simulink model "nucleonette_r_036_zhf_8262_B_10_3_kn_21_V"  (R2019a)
settings: Solver=VariableStepAuto  StartTime=0.0  StopTime=727544.216  FixedStep=0.2  RelTol=1e-6
libraries: simulink x6
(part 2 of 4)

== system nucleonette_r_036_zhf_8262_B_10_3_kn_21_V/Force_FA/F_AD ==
  In1 : Inport
  In2 : Inport  Port=2
  Add21 : Sum  Inputs=+-
  Add27 : Sum  Inputs=-+++
  Add32 : Sum  Inputs=+++
  Add35 : Sum
  Add38 : Sum  Inputs=++++
  Add53 : Sum
  C_100_1 : Constant  Value=-100
  C_10_1 : Constant  Value=10
  C_10_11_2 : Constant  Value=1E-21
  Clock1 : Clock
  Constant : Constant
  Constant1 : Constant  Value=2
  Constant13 : Constant  Value=3
  Constant15 : Constant  Value=1.0E-3
  Constant19 : Constant  Value=2
  Constant24 : Constant  Value=3
  Constant26 : Constant  Value=3
  Math Function{17,24,34,36} (4 alike) : Math  Operator=square
  Math Function35 : Math  Operator=pow
  Math Function39 : Math  Operator=pow
  Math Function45 : Math  Operator=pow
  Nadx/Dadx : Scope
  Omega_w1 : Constant  Value=0.00003453723537
  Product{1..4,27,54..56,66} (9 alike) : Product  Inputs=**
  Product{29,46,50,57} (4 alike) : Product
  Product40 : Product  Inputs=*/
  Product48 : Product  Inputs=/**
  Product5 : Product  Inputs=/*
  Product62 : Product  Inputs=*/
  Product63 : Product  Inputs=/*
  Product65 : Product  Inputs=*/*
  Sqrt10 : Sqrt
  Sqrt14 : Sqrt
  Trigonometric Function11 : Trigonometry
  Trigonometric Function12 : Trigonometry  Operator=cos
  Trigonometric Function7 : Trigonometry
  Trigonometric Function8 : Trigonometry  Operator=cos
  ex : Constant  Value=1.602176565
  kADx : Constant  Value=66.535517341
  mFAx : Constant  Value=999.755388642
  rx1 : Constant  Value=0.36373
  Out1 : Outport
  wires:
  Product57/1 -> Trigonometric Function12/1, Product29/2, Trigonometric Function11/1
  Math Function34/1 -> Add32/3  "Zad_2"
  kADx/1 -> Product48/3
  rx1/1 -> Product27/1, Product5/2, Product54/1, Product4/1, Product65/2, Product56/1, Product55/1  "rx"
  In2/1 -> Product1/1  "z4"
  Math Function17/1 -> Add32/1  "Yad_2"
  C_10_11_2/1 -> Add35/2
  Product40/1 -> Nadx/Dadx/1, Out1/1  "nad/dad"
  Omega_w1/1 -> Product57/2
  Add32/1 -> Sqrt10/1  "Dad_2"
  Constant13/1 -> Product29/1, Sqrt14/1
  Product66/1 -> Product50/2  "kn_Dad"
  Add53/1 -> Product40/2  "Dad_B"
  Math Function36/1 -> Add32/2  "Xad_2"
  Product54/1 -> Add21/1  "r*cos(3wt)"
  Product63/1 -> Product3/2, Product1/2  "1/2"
  Add38/1 -> Math Function17/1  "YAD"
  Add27/1 -> Math Function34/1, Product50/1  "ZAD"
  C_10_1/1 -> Math Function39/1
  Product65/1 -> Math Function39/2
  Product29/1 -> Trigonometric Function8/1, Trigonometric Function7/1
  Product62/1 -> Add38/1  "r*sin(3wt)/2"
  Constant1/1 -> Product63/1
  Product50/1 -> Product40/1  "Nad"
  Math Function39/1 -> Add35/1  "10_exp(-100Dad/r)"
  Constant24/1 -> Math Function45/2
  Math Function45/1 -> Add53/1
  Add21/1 -> Math Function36/1  "XAD"
  In1/1 -> Add27/2  "z0 - z + delta"
  ex/1 -> Math Function24/1
  Constant19/1 -> Product62/2, Product5/1  "2"
  Math Function24/1 -> Product48/2
  Sqrt10/1 -> Product65/1, Math Function35/1  "Dad"
  Constant/1 -> Product63/2
  Trigonometric Function11/1 -> Product55/2  "sin(wt)"
  Trigonometric Function12/1 -> Product56/2  "cos(wt)"
  Product2/1 -> Add38/3  "z4*sqrt(3)/2"
  Add35/1 -> Product66/1
  Constant26/1 -> Math Function35/2
  Clock1/1 -> Product57/1
  Product27/1 -> Product46/1, Product62/1  "r*sin(3wt)"
  Product48/1 -> Product66/2
  Math Function35/1 -> Add53/2  "Dad_3"
  Sqrt14/1 -> Product3/1, Product2/1  "sqrt(3)"
  mFAx/1 -> Product48/1  "mx"
  Constant15/1 -> Math Function45/1
  C_100_1/1 -> Product65/3
  Product56/1 -> Add21/2  "r*cos(wt)"
  Trigonometric Function8/1 -> Product54/2  "cos(3wt)"
  Product3/1 -> Product46/2, Product4/2  "sqrt(3)/2"
  Trigonometric Function7/1 -> Product27/2  "sin(3wt)"
  Product5/1 -> Add38/2  "r/2"
  Product1/1 -> Product2/2, Add27/3  "z4/2"
  Product4/1 -> Add27/4  "r*sqrt(3)/2"
  Product55/1 -> Add38/4  "r*sin(wt)"
  Product46/1 -> Add27/1  "r*sin(3wt)*sqrt(3)/2"

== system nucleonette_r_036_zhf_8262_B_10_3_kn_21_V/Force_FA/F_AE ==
  In1 : Inport
  In2 : Inport  Port=2
  Add21 : Sum  Inputs=--
  Add27 : Sum  Inputs=++++
  Add32 : Sum  Inputs=+++
  Add35 : Sum
  Add38 : Sum  Inputs=-+++
  Add53 : Sum
  C_100_1 : Constant  Value=-100
  C_10_1 : Constant  Value=10
  C_10_11_2 : Constant  Value=1E-21
  Clock1 : Clock
  Constant : Constant
  Constant1 : Constant  Value=2
  Constant13 : Constant  Value=3
  Constant15 : Constant  Value=1.0E-3
  Constant19 : Constant  Value=2
  Constant24 : Constant  Value=3
  Constant26 : Constant  Value=3
  Math Function{17,24,34,36} (4 alike) : Math  Operator=square
  Math Function35 : Math  Operator=pow
  Math Function39 : Math  Operator=pow
  Math Function45 : Math  Operator=pow
  Naex/Daex : Scope
  Omega_w1 : Constant  Value=0.00003453723537
  Product{1..4,27,54..56,66} (9 alike) : Product  Inputs=**
  Product{29,46,50,57} (4 alike) : Product
  Product40 : Product  Inputs=*/
  Product48 : Product  Inputs=/**
  Product5 : Product  Inputs=/*
  Product62 : Product  Inputs=*/
  Product63 : Product  Inputs=/*
  Product65 : Product  Inputs=*/*
  Sqrt10 : Sqrt
  Sqrt14 : Sqrt
  Trigonometric Function11 : Trigonometry
  Trigonometric Function12 : Trigonometry  Operator=cos
  Trigonometric Function7 : Trigonometry
  Trigonometric Function8 : Trigonometry  Operator=cos
  ex : Constant  Value=1.602176565
  kAEx : Constant  Value=66.535517341
  mFAx : Constant  Value=999.755388642
  rx1 : Constant  Value=0.36373
  Out1 : Outport
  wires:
  Add38/1 -> Math Function17/1  "YAE"
  Math Function36/1 -> Add32/2  "Xae_2"
  mFAx/1 -> Product48/1  "mx"
  Constant15/1 -> Math Function45/1
  C_100_1/1 -> Product65/3
  Sqrt14/1 -> Product3/1, Product2/1  "sqrt(3)"
  Product55/1 -> Add38/4  "r*sin(wt)"
  Product4/1 -> Add27/4  "r*sqrt(3)/2"
  Math Function39/1 -> Add35/1  "10_exp(-100Dae/r)"
  Constant1/1 -> Product63/1
  Product50/1 -> Product40/1  "Nae"
  Product54/1 -> Add21/1  "r*cos(3wt)"
  Product3/1 -> Product46/2, Product4/2  "sqrt(3)/2"
  Product48/1 -> Product66/2
  Product1/1 -> Product2/2, Add27/3  "z4/2"
  In1/1 -> Add27/2  "z0 - z + delta"
  Add21/1 -> Math Function36/1  "XAE"
  Trigonometric Function11/1 -> Product55/2  "sin(wt)"
  Add35/1 -> Product66/1
  Math Function35/1 -> Add53/2  "Dae_3"
  Trigonometric Function8/1 -> Product54/2  "cos(3wt)"
  Math Function24/1 -> Product48/2
  Product56/1 -> Add21/2  "r*cos(wt)"
  Trigonometric Function7/1 -> Product27/2  "sin(3wt)"
  Constant19/1 -> Product62/2, Product5/1  "2"
  Constant/1 -> Product63/2
  Product2/1 -> Add38/3  "z4*sqrt(3)/2"
  Trigonometric Function12/1 -> Product56/2  "cos(wt)"
  Clock1/1 -> Product57/1
  Constant26/1 -> Math Function35/2
  Product29/1 -> Trigonometric Function8/1, Trigonometric Function7/1
  Product46/1 -> Add27/1  "r*sin(3wt)*sqrt(3)/2"
  Product65/1 -> Math Function39/2
  C_10_1/1 -> Math Function39/1
  Constant24/1 -> Math Function45/2
  ex/1 -> Math Function24/1
  Product57/1 -> Trigonometric Function12/1, Product29/2, Trigonometric Function11/1
  Math Function34/1 -> Add32/3  "Zae_2"
  Product63/1 -> Product3/2, Product1/2  "1/2"
  Product5/1 -> Add38/2  "r/2"
  Add27/1 -> Math Function34/1, Product50/1  "ZAE"
  Omega_w1/1 -> Product57/2
  Constant13/1 -> Product29/1, Sqrt14/1
  Add32/1 -> Sqrt10/1  "Dae_2"
  Product40/1 -> Naex/Daex/1, Out1/1  "nae/dae"
  Product27/1 -> Product46/1, Product62/1  "r*sin(3wt)"
  Math Function45/1 -> Add53/1
  Product66/1 -> Product50/2  "kn_Dae"
  Product62/1 -> Add38/1  "r*sin(3wt)/2"
  kAEx/1 -> Product48/3
  Add53/1 -> Product40/2  "Dae_B"
  rx1/1 -> Product27/1, Product5/2, Product54/1, Product4/1, Product65/2, Product56/1, Product55/1  "rx"
  Sqrt10/1 -> Product65/1, Math Function35/1  "Dae"
  C_10_11_2/1 -> Add35/2
  Math Function17/1 -> Add32/1  "Yae_2"
  In2/1 -> Product1/1  "z4"

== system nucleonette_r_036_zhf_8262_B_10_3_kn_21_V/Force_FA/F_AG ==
  In1 : Inport
  In2 : Inport  Port=2
  Add28 : Sum  Inputs=+-
  Add29 : Sum  Inputs=-++
  Add30 : Sum  Inputs=+++
  Add34 : Sum  Inputs=+++
  Add36 : Sum
  Add54 : Sum
  C_100_1 : Constant  Value=-100
  C_10_1 : Constant  Value=10
  C_10_11_2 : Constant  Value=1E-21
  Clock1 : Clock
  Constant{13,24..26} (4 alike) : Constant  Value=3
  Constant15 : Constant  Value=1.0E-3
  Constant19 : Constant  Value=2
  Constant23 : Constant  Value=2
  Math Function{21,24,26,31} (4 alike) : Math  Operator=square
  Math Function23 : Math  Operator=pow
  Math Function40 : Math  Operator=pow
  Math Function45 : Math  Operator=pow
  Nagx/Dagx_3 : Scope
  Omega_w1 : Constant  Value=0.00003453723537
  Product{27,55..56,62,67} (5 alike) : Product  Inputs=**
  Product{29,46,52,57} (4 alike) : Product
  Product47 : Product  Inputs=*/
  Product48 : Product  Inputs=/**
  Product54 : Product  Inputs=**/
  Product63 : Product  Inputs=/*
  Product64 : Product  Inputs=*/*
  Sqrt13 : Sqrt
  Sqrt14 : Sqrt
  Sqrt15 : Sqrt
  Trigonometric Function11 : Trigonometry
  Trigonometric Function12 : Trigonometry  Operator=cos
  Trigonometric Function7 : Trigonometry
  Trigonometric Function8 : Trigonometry  Operator=cos
  ex : Constant  Value=1.602176565
  k16x1 : Constant  Value=66.535517341
  mFAx : Constant  Value=999.755388642
  rx1 : Constant  Value=0.36373
  Out1 : Outport
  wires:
  Product52/1 -> Product47/1  "Nag"
  Product29/1 -> Trigonometric Function8/1, Trigonometric Function7/1
  C_10_11_2/1 -> Add36/1
  Constant13/1 -> Sqrt13/1
  Add54/1 -> Product47/2  "Dag_B"
  Constant15/1 -> Math Function45/1
  Add29/1 -> Math Function21/1  "X3a"
  Constant25/1 -> Sqrt14/1, Product29/2
  Add34/1 -> Sqrt15/1  "Dag_2"
  Constant24/1 -> Math Function45/2
  Trigonometric Function11/1 -> Product55/2  "sin(wt)"
  Product54/1 -> Add29/3, Product46/1  "r*cos(3wt)/2"
  Constant23/1 -> Product54/3
  Product48/1 -> Product67/2
  Trigonometric Function12/1 -> Product56/2  "cos(wt)"
  Math Function40/1 -> Add36/2  "10_exp(-100Dag/r)"
  Product64/1 -> Math Function40/2
  Trigonometric Function7/1 -> Product27/2  "sin(3wt)"
  Product47/1 -> Out1/1, Nagx/Dagx_3/1  "Nag/Dag_3"
  ex/1 -> Math Function24/1
  Product62/1 -> Add29/1  "(z0 - z3)*sqrt(3)/2"
  Product55/1 -> Add28/2  "r*sin(wt)"
  Clock1/1 -> Product57/1
  Product27/1 -> Add28/1  "r*sin(3wt)"
  Constant26/1 -> Math Function23/2
  Sqrt14/1 -> Product46/2  "sqrt(3)"
  Sqrt13/1 -> Product62/1  "sqrt(3)"
  Product57/1 -> Trigonometric Function12/1, Trigonometric Function11/1, Product29/1
  Math Function45/1 -> Add54/1
  Math Function23/1 -> Add54/2  "Dag_3"
  Constant19/1 -> Product63/1  "2"
  C_100_1/1 -> Product64/1
  Trigonometric Function8/1 -> Product54/2  "cos(3wt)"
  Product67/1 -> Product52/2  "kn_Dag"
  Sqrt15/1 -> Math Function23/1, Product64/3  "Dag"
  Product56/1 -> Add29/2  "r*cos(wt)"
  Add28/1 -> Math Function31/1  "r*sin(3wt) - r*sin(wt)"
  C_10_1/1 -> Math Function40/1
  Product46/1 -> Add30/1  "r*cos(3wt)*sqrt(3)/2"
  Product63/1 -> Add30/2, Product62/2  "(z0 - z3)/2"
  Math Function24/1 -> Product48/2
  Add36/1 -> Product67/1
  Omega_w1/1 -> Product57/2
  k16x1/1 -> Product48/3
  Math Function26/1 -> Add34/3  "Zag_2"
  mFAx/1 -> Product48/1  "mx"
  Math Function21/1 -> Add34/2  "Xag_2"
  Math Function31/1 -> Add34/1  "Yag_2"
  rx1/1 -> Product56/1, Product55/1, Product27/1, Product54/1, Product64/2  "rx"
  In2/1 -> Product63/2
  Add30/1 -> Math Function26/1, Product52/1  "Z3f"
  In1/1 -> Add30/3

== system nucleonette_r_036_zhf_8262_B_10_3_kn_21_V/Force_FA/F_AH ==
  In1 : Inport
  In2 : Inport  Port=2
  Add21 : Sum  Inputs=++-
  Add27 : Sum  Inputs=+--
  Add32 : Sum  Inputs=+++
  Add35 : Sum
  Add38 : Sum
  Add53 : Sum
  C_100_1 : Constant  Value=-100
  C_10_1 : Constant  Value=10
  C_10_11_2 : Constant  Value=1E-21
  Clock1 : Clock
  Constant13 : Constant  Value=3
  Constant15 : Constant  Value=1.0E-3
  Constant18 : Constant  Value=1E-17
  Constant19 : Constant  Value=2
  Constant20 : Constant  Value=-2E-17
  Constant23 : Constant  Value=2
  Constant24 : Constant  Value=3
  Constant26 : Constant  Value=3
  Logical Operator3 : Logic  AllPortsSameDT=off  OutDataTypeStr=boolean
  Math Function{17,24,34,36} (4 alike) : Math  Operator=square
  Math Function35 : Math  Operator=pow
  Math Function39 : Math  Operator=pow
  Math Function45 : Math  Operator=pow
  Nahx/Dahx_1 : Scope
  Nahx/Dahx_3 : Scope
  Omega_w1 : Constant  Value=0.00003453723537
  Product{27,55..56,62,66} (5 alike) : Product  Inputs=**
  Product{29,46,50,57,76} (5 alike) : Product
  Product40 : Product  Inputs=*/
  Product48 : Product  Inputs=/**
  Product54 : Product  Inputs=**/
  Product63 : Product  Inputs=/*
  Product65 : Product  Inputs=*/*
  Relational Operator3 : RelationalOperator  Operator=>  OutDataTypeStr=boolean  RndMeth=Simplest
  Relational Operator7 : RelationalOperator  Operator=<  OutDataTypeStr=boolean  RndMeth=Simplest
  Sqrt10 : Sqrt
  Sqrt13 : Sqrt
  Sqrt14 : Sqrt
  Trigonometric Function11 : Trigonometry
  Trigonometric Function12 : Trigonometry  Operator=cos
  Trigonometric Function7 : Trigonometry
  Trigonometric Function8 : Trigonometry  Operator=cos
  ex : Constant  Value=1.602176565
  kAHx : Constant  Value=66.535517341
  mFAx : Constant  Value=999.755388642
  rx1 : Constant  Value=0.36373
  Out1 : Outport
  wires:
  Product50/1 -> Product40/1  "Nah"
  C_10_1/1 -> Math Function39/1
  Constant26/1 -> Math Function35/2
  Product27/1 -> Add38/1  "r*sin(3wt)"
  Product46/1 -> Add27/1  "r*cos(3wt)*sqrt(3)/2"
  Product65/1 -> Math Function39/2
  Math Function36/1 -> Add32/2  "Xah_2"
  Sqrt10/1 -> Product65/1, Math Function35/1  "Dah"
  Math Function24/1 -> Product48/2
  mFAx/1 -> Product48/1  "mx"
  Math Function17/1 -> Add32/1  "Yah_2"
  ex/1 -> Math Function24/1
  kAHx/1 -> Product48/3
  Add53/1 -> Product40/2  "Dah_B"
  Logical Operator3/1 -> Product76/2
  Add27/1 -> Math Function34/1, Product50/1  "Z2a"
  Product54/1 -> Add21/2, Product46/1  "r*cos(3wt)/2"
  Product76/1 -> Nahx/Dahx_1/1  "Fah_1"
  C_100_1/1 -> Product65/3
  Add38/1 -> Math Function17/1  "r*sin(3wt) + r*sin(wt)"
  Product55/1 -> Add38/2  "r*sin(wt)"
  Add32/1 -> Sqrt10/1  "Dah_2"
  Sqrt14/1 -> Product46/2  "sqrt(3)"
  Product62/1 -> Add21/1  "(z0 - z3)*sqrt(3)/2"
  Constant19/1 -> Product63/1  "2"
  Constant13/1 -> Product29/1, Sqrt14/1, Sqrt13/1
  Constant15/1 -> Math Function45/1
  Constant18/1 -> Relational Operator3/1
  Product63/1 -> Add27/2, Product62/2  "(z0 - z3)/2"
  Add35/1 -> Product66/1
  Sqrt13/1 -> Product62/1  "sqrt(3)"
  Math Function34/1 -> Add32/3  "Zah_2"
  Product29/1 -> Trigonometric Function8/1, Trigonometric Function7/1
  Add21/1 -> Math Function36/1  "X2a"
  Constant24/1 -> Math Function45/2
  Trigonometric Function11/1 -> Product55/2  "sin(wt)"
  Constant23/1 -> Product54/3
  Trigonometric Function8/1 -> Product54/2  "cos(3wt)"
  Trigonometric Function12/1 -> Product56/2  "cos(wt)"
  Constant20/1 -> Relational Operator7/1
  rx1/1 -> Product27/1, Product54/1, Product65/2, Product56/1, Product55/1  "rx"
  Trigonometric Function7/1 -> Product27/2  "sin(3wt)"
  Relational Operator7/1 -> Logical Operator3/2
  Relational Operator3/1 -> Logical Operator3/1
  Math Function39/1 -> Add35/1  "10_exp(-100Dah/r)"
  Product56/1 -> Add21/3  "r*cos(wt)"
  Product48/1 -> Product66/2
  C_10_11_2/1 -> Add35/2
  Math Function35/1 -> Add53/2  "Dah_3"
  Product66/1 -> Product50/2  "kn_Dah"
  In2/1 -> Product63/2
  In1/1 -> Add27/3
  Math Function45/1 -> Add53/1
  Clock1/1 -> Product57/1
  Product57/1 -> Trigonometric Function12/1, Product29/2, Trigonometric Function11/1
  Omega_w1/1 -> Product57/2
  Product40/1 -> Nahx/Dahx_3/1, Product76/1, Relational Operator3/2, Relational Operator7/2, Out1/1  "nah/dah_3"

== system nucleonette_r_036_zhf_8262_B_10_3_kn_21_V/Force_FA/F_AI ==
  In1 : Inport
  Add12 : Sum  Inputs=-+
  Add33 : Sum  Inputs=--
  Add37 : Sum
  Add39 : Sum
  Add52 : Sum
  C_10 : Constant  Value=10
  C_100 : Constant  Value=-100
  C_10_11 : Constant  Value=1E-21
  Clock1 : Clock
  Constant10 : Constant  Value=0.86602
  Constant13 : Constant  Value=3
  Constant15 : Constant  Value=1.0E-3
  Constant19 : Constant  Value=2
  Constant21 : Constant  Value=1.5
  Constant24 : Constant  Value=3
  Math Function25 : Math  Operator=square
  Math Function28 : Math  Operator=square
  Math Function33 : Math  Operator=pow
  Math Function38 : Math  Operator=pow
  Math Function4 : Math  Operator=square
  Math Function45 : Math  Operator=pow
  Naix/Daix_3 : Scope
  Omega_w1 : Constant  Value=0.00003453723537
  Product25 : Product  Inputs=**/
  Product28 : Product  Inputs=*/
  Product31 : Product  Inputs=/**
  Product{32,53,57,59,61} (5 alike) : Product
  Product44 : Product  Inputs=**/
  Product51 : Product  Inputs=*/*
  Product58 : Product  Inputs=3
  Sqrt11 : Sqrt
  Sqrt13 : Sqrt
  Trigonometric Function10 : Trigonometry  Operator=cos
  ex : Constant  Value=1.602176565
  kAIx : Constant  Value=7.39283526
  mAIx : Constant  Value=999.755388642
  rx1 : Constant  Value=0.36373
  Out1 : Outport
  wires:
  Sqrt11/1 -> Product51/3, Math Function33/1  "Dai"
  Constant13/1 -> Sqrt13/1, Product32/2
  Constant15/1 -> Math Function45/1
  Product25/1 -> Product32/1  "r*cos(wt)/2"
  Add33/1 -> Math Function25/1
  kAIx/1 -> Product31/3
  Product59/1 -> Add12/1  "3*z/2"
  Add12/1 -> Math Function28/1, Product61/2  "Zai"
  Product32/1 -> Add33/2  "3r*cos(wt)/2"
  Product61/1 -> Product28/1
  Constant24/1 -> Math Function33/2, Math Function45/2
  Add52/1 -> Product28/2  "Dai_B"
  C_10_11/1 -> Add39/1
  Add39/1 -> Product53/1  "kn_Dai"
  Math Function25/1 -> Add37/2
  Math Function28/1 -> Add37/1
  Math Function4/1 -> Product31/2
  Clock1/1 -> Product57/1
  Product58/1 -> Add12/2  "r*cos(wt)*sqrt(3)/2"
  Sqrt13/1 -> Product44/2  "sqrt(3)"
  C_100/1 -> Product51/1
  Product57/1 -> Trigonometric Function10/1  "angle_wt"
  Product44/1 -> Add33/1  "z*sqrt(3)/2"
  Math Function45/1 -> Add52/1
  Math Function33/1 -> Add52/2
  ex/1 -> Math Function4/1
  Constant19/1 -> Product25/3, Product44/3  "2"
  Trigonometric Function10/1 -> Product58/2, Product25/1  "cos(wt)"
  Constant10/1 -> Product58/1  "sqrt(3)/2"
  Product53/1 -> Product61/1
  Product28/1 -> Out1/1, Naix/Daix_3/1  "naix/daix_3"
  Omega_w1/1 -> Product57/2
  Add37/1 -> Sqrt11/1
  C_10/1 -> Math Function38/1
  Math Function38/1 -> Add39/2  "10_exp(-100Dai/r)"
  Product51/1 -> Math Function38/2
  rx1/1 -> Product51/2, Product58/3, Product25/2  "rx"
  mAIx/1 -> Product31/1  "mx"
  Product31/1 -> Product53/2
  In1/1 -> Product59/2, Product44/1
  Constant21/1 -> Product59/1

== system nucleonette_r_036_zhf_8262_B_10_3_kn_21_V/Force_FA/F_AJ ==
  In1 : Inport
  Add31 : Sum  Inputs=+++
  Add40 : Sum
  Add51 : Sum
  C_10 : Constant  Value=10
  C_100 : Constant  Value=-100
  C_10_11 : Constant  Value=1E-21
  Clock1 : Clock
  Constant13 : Constant  Value=3
  Constant14 : Constant  Value=2
  Constant15 : Constant  Value=1.0E-3
  Constant17 : Constant  Value=1E-22
  Constant19 : Constant  Value=2
  Constant21 : Constant  Value=1.5
  Constant24 : Constant  Value=3
  Math Function{4,27,29..30} (4 alike) : Math  Operator=square
  Math Function32 : Math  Operator=pow
  Math Function37 : Math  Operator=pow
  Math Function45 : Math  Operator=pow
  Najx/Dajx_1 : Scope
  Najx/Dajx_3 : Scope
  Omega_w1 : Constant  Value=0.00003453723537
  Product{12,20,45,57,59..60,75} (7 alike) : Product
  Product25 : Product  Inputs=**/
  Product26 : Product  Inputs=*/
  Product31 : Product  Inputs=/**
  Product33 : Product  Inputs=/**
  Product44 : Product  Inputs=**/
  Product58 : Product  Inputs=3
  Relational Operator1 : RelationalOperator  Operator=>  OutDataTypeStr=boolean  RndMeth=Simplest
  Sqrt13 : Sqrt
  Sqrt4 : Sqrt
  Subtract3 : Sum
  Subtract4 : Sum  Inputs=--
  Trigonometric Function10 : Trigonometry  Operator=cos
  Trigonometric Function9 : Trigonometry
  ex : Constant  Value=1.602176565
  kAJx : Constant  Value=7.39283526
  mFAx : Constant  Value=999.755388642
  rx1 : Constant  Value=0.36373
  sqrt(3)/2 : Constant  Value=0.86602
  Out1 : Outport
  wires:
  Subtract4/1 -> Math Function30/1
  Math Function32/1 -> Add51/2
  Add40/1 -> Product45/1  "kn_Daj"
  Math Function45/1 -> Add51/1
  Product45/1 -> Product60/1
  Math Function4/1 -> Product31/2
  Math Function30/1 -> Add31/3
  Math Function37/1 -> Add40/1  "10_exp(-100Daj/r)"
  Product75/1 -> Najx/Dajx_1/1  "Faj_1"
  Math Function29/1 -> Add31/2
  Clock1/1 -> Product57/1
  Product44/1 -> Subtract4/1  "z*sqrt(3)/2"
  sqrt(3)/2/1 -> Product58/1  "sqrt(3)/2"
  Subtract3/1 -> Math Function27/1, Product60/2  "Zaj"
  Constant17/1 -> Relational Operator1/1
  C_100/1 -> Product33/3
  Trigonometric Function10/1 -> Product58/2, Product25/1  "cos(wt)"
  Product58/1 -> Subtract3/2  "r*cos(wt)*sqrt(3)/2"
  Add51/1 -> Product26/2  "Daj_B"
  Add31/1 -> Sqrt4/1
  C_10_11/1 -> Add40/2
  Relational Operator1/1 -> Product75/1
  Product31/1 -> Product45/2
  Constant21/1 -> Product59/2
  Product57/1 -> Trigonometric Function9/1, Trigonometric Function10/1  "angle_wt"
  C_10/1 -> Math Function37/1
  mFAx/1 -> Product31/1  "mx"
  Constant19/1 -> Product25/3, Product44/3  "2"
  Constant13/1 -> Sqrt13/1
  Product33/1 -> Math Function37/2
  Constant15/1 -> Math Function45/1
  Product59/1 -> Subtract3/1  "3*z/2"
  Omega_w1/1 -> Product57/2
  Sqrt13/1 -> Product44/2  "sqrt(3)"
  kAJx/1 -> Product31/3
  ex/1 -> Math Function4/1
  Product12/1 -> Product20/2  "r*sin(wt)"
  Math Function27/1 -> Add31/1
  Constant24/1 -> Math Function32/2, Math Function45/2
  Constant14/1 -> Product20/1
  Trigonometric Function9/1 -> Product12/1  "sin(wt)"
  Product25/1 -> Subtract4/2  "r*cos(wt)/2"
  rx1/1 -> Product33/1, Product25/2, Product12/2, Product58/3  "rx"
  Product20/1 -> Math Function29/1  "2r*sin(wt)"
  Product26/1 -> Out1/1, Product75/2, Relational Operator1/2, Najx/Dajx_3/1  "F_AJ"
  Sqrt4/1 -> Product33/2, Math Function32/1  "Daj"
  In1/1 -> Product44/1, Product59/1  "z"
  Product60/1 -> Product26/1

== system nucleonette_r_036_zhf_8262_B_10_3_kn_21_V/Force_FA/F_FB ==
  In1 : Inport
  In2 : Inport  Port=2
  Add21 : Sum
  Add27 : Sum  Inputs=++++
  Add32 : Sum  Inputs=+++
  Add35 : Sum
  Add38 : Sum  Inputs=+---
  Add53 : Sum
  C_100_1 : Constant  Value=-100
  C_10_1 : Constant  Value=10
  C_10_11_2 : Constant  Value=1E-21
  Clock1 : Clock
  Constant : Constant
  Constant1 : Constant  Value=2
  Constant13 : Constant  Value=3
  Constant15 : Constant  Value=1.0E-3
  Constant19 : Constant  Value=2
  Constant24 : Constant  Value=3
  Constant26 : Constant  Value=3
  Math Function{17,24,34,36} (4 alike) : Math  Operator=square
  Math Function35 : Math  Operator=pow
  Math Function39 : Math  Operator=pow
  Math Function45 : Math  Operator=pow
  Nfbx/Dfbx : Scope
  Omega_w1 : Constant  Value=0.00003453723537
  Product{1..4,27,54..56,66} (9 alike) : Product  Inputs=**
  Product{29,46,50,57} (4 alike) : Product
  Product40 : Product  Inputs=*/
  Product48 : Product  Inputs=/**
  Product5 : Product  Inputs=/*
  Product62 : Product  Inputs=*/
  Product63 : Product  Inputs=/*
  Product65 : Product  Inputs=*/*
  Sqrt10 : Sqrt
  Sqrt14 : Sqrt
  Trigonometric Function11 : Trigonometry
  Trigonometric Function12 : Trigonometry  Operator=cos
  Trigonometric Function7 : Trigonometry
  Trigonometric Function8 : Trigonometry  Operator=cos
  ex : Constant  Value=1.602176565
  kFBx : Constant  Value=66.535517341
  mFAx : Constant  Value=999.755388642
  rx1 : Constant  Value=0.36373
  Out1 : Outport
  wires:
  Product40/1 -> Nfbx/Dfbx/1, Out1/1  "nfb/dfb"
  Product57/1 -> Trigonometric Function12/1, Product29/2, Trigonometric Function11/1
  Add27/1 -> Math Function34/1, Product50/1  "ZFB"
  ex/1 -> Math Function24/1
  Product56/1 -> Add21/2  "r*cos(wt)"
  Omega_w1/1 -> Product57/2
  Math Function35/1 -> Add53/2  "Dfb_3"
  Math Function45/1 -> Add53/1
  Add21/1 -> Math Function36/1  "XFB"
  Constant24/1 -> Math Function45/2
  C_10_11_2/1 -> Add35/2
  Product48/1 -> Product66/2
  Math Function39/1 -> Add35/1  "10_exp(-100Dfb/r)"
  Math Function24/1 -> Product48/2
  Trigonometric Function7/1 -> Product27/2  "sin(3wt)"
  rx1/1 -> Product27/1, Product5/2, Product54/1, Product4/1, Product65/2, Product56/1, Product55/1  "rx"
  Trigonometric Function12/1 -> Product56/2  "cos(wt)"
  Constant15/1 -> Math Function45/1
  Trigonometric Function8/1 -> Product54/2  "cos(3wt)"
  Trigonometric Function11/1 -> Product55/2  "sin(wt)"
  Math Function34/1 -> Add32/3  "Zfb_2"
  Add35/1 -> Product66/1
  Product29/1 -> Trigonometric Function8/1, Trigonometric Function7/1
  Product46/1 -> Add27/1  "r*sin(3wt)*sqrt(3)/2"
  Constant13/1 -> Product29/1, Sqrt14/1
  Add32/1 -> Sqrt10/1  "Dfb_2"
  Product27/1 -> Product46/1, Product62/1  "r*sin(3wt)"
  Add38/1 -> Math Function17/1  "YFB"
  C_100_1/1 -> Product65/3
  mFAx/1 -> Product48/1  "mx"
  Product66/1 -> Product50/2  "kn_Dfb"
  Clock1/1 -> Product57/1
  kFBx/1 -> Product48/3
  Add53/1 -> Product40/2  "Dfb_B"
  Math Function17/1 -> Add32/1  "Yfb_2"
  Sqrt10/1 -> Product65/1, Math Function35/1  "Dfb"
  Math Function36/1 -> Add32/2  "Xfb_2"
  Product65/1 -> Math Function39/2
  Constant26/1 -> Math Function35/2
  C_10_1/1 -> Math Function39/1
  Product50/1 -> Product40/1  "Nfb"
  In2/1 -> Product1/1  "z4"
  Constant1/1 -> Product63/1
  Product1/1 -> Product2/2, Add27/3  "z4/2"
  In1/1 -> Add27/2  "z0 - z + delta"
  Constant/1 -> Product63/2
  Product63/1 -> Product3/2, Product1/2  "1/2"
  Sqrt14/1 -> Product3/1, Product2/1  "sqrt(3)"
  Product3/1 -> Product46/2, Product4/2  "sqrt(3)/2"
  Product4/1 -> Add27/4  "r*sqrt(3)/2"
  Product54/1 -> Add21/1  "r*cos(3wt)"
  Product55/1 -> Add38/4  "r*sin(wt)"
  Product62/1 -> Add38/1  "r*sin(3wt)/2"
  Product2/1 -> Add38/3  "z4*sqrt(3)/2"
  Constant19/1 -> Product62/2, Product5/1  "2"
  Product5/1 -> Add38/2  "r/2"

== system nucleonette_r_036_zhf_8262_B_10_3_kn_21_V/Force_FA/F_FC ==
  In1 : Inport
  In2 : Inport  Port=2
  Add21 : Sum  Inputs=-+
  Add27 : Sum  Inputs=-+++
  Add32 : Sum  Inputs=+++
  Add35 : Sum
  Add38 : Sum  Inputs=----
  Add53 : Sum
  C_100_1 : Constant  Value=-100
  C_10_1 : Constant  Value=10
  C_10_11_2 : Constant  Value=1E-21
  Clock1 : Clock
  Constant : Constant
  Constant1 : Constant  Value=2
  Constant13 : Constant  Value=3
  Constant15 : Constant  Value=1.0E-3
  Constant19 : Constant  Value=2
  Constant24 : Constant  Value=3
  Constant26 : Constant  Value=3
  Math Function{17,24,34,36} (4 alike) : Math  Operator=square
  Math Function35 : Math  Operator=pow
  Math Function39 : Math  Operator=pow
  Math Function45 : Math  Operator=pow
  Nfcx/Dfcx : Scope
  Omega_w1 : Constant  Value=0.00003453723537
  Product{1..4,27,54..56,66} (9 alike) : Product  Inputs=**
  Product{29,46,50,57} (4 alike) : Product
  Product40 : Product  Inputs=*/
  Product48 : Product  Inputs=/**
  Product5 : Product  Inputs=/*
  Product62 : Product  Inputs=*/
  Product63 : Product  Inputs=/*
  Product65 : Product  Inputs=*/*
  Sqrt10 : Sqrt
  Sqrt14 : Sqrt
  Trigonometric Function11 : Trigonometry
  Trigonometric Function12 : Trigonometry  Operator=cos
  Trigonometric Function7 : Trigonometry
  Trigonometric Function8 : Trigonometry  Operator=cos
  ex : Constant  Value=1.602176565
  kFCx : Constant  Value=66.535517341
  mFAx : Constant  Value=999.755388642
  rx1 : Constant  Value=0.36373
  Out1 : Outport
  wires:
  Product2/1 -> Add38/3  "z4*sqrt(3)/2"
  In2/1 -> Product1/1  "z4"
  Product56/1 -> Add21/2  "r*cos(wt)"
  C_10_1/1 -> Math Function39/1
  Math Function34/1 -> Add32/3  "Zfc_2"
  Clock1/1 -> Product57/1
  Trigonometric Function12/1 -> Product56/2  "cos(wt)"
  Constant26/1 -> Math Function35/2
  Product46/1 -> Add27/1  "r*sin(3wt)*sqrt(3)/2"
  Product65/1 -> Math Function39/2
  Constant15/1 -> Math Function45/1
  C_100_1/1 -> Product65/3
  Math Function36/1 -> Add32/2  "Xfc_2"
  mFAx/1 -> Product48/1  "mx"
  Add38/1 -> Math Function17/1  "YFC"
  Sqrt10/1 -> Product65/1, Math Function35/1  "Dfc"
  C_10_11_2/1 -> Add35/2
  Math Function17/1 -> Add32/1  "Yfc_2"
  Add53/1 -> Product40/2  "Dfc_B"
  kFCx/1 -> Product48/3
  Product66/1 -> Product50/2  "kn_Dfc"
  Product29/1 -> Trigonometric Function8/1, Trigonometric Function7/1
  Product27/1 -> Product46/1, Product62/1  "r*sin(3wt)"
  Add32/1 -> Sqrt10/1  "Dfc_2"
  Product40/1 -> Nfcx/Dfcx/1, Out1/1  "nfc/dfc"
  Omega_w1/1 -> Product57/2
  Constant13/1 -> Product29/1, Sqrt14/1
  Add35/1 -> Product66/1
  Add21/1 -> Math Function36/1  "XFC"
  Trigonometric Function11/1 -> Product55/2  "sin(wt)"
  Trigonometric Function8/1 -> Product54/2  "cos(3wt)"
  Math Function35/1 -> Add53/2  "Dfc_3"
  Math Function24/1 -> Product48/2
  rx1/1 -> Product27/1, Product5/2, Product54/1, Product4/1, Product65/2, Product56/1, Product55/1  "rx"
  Trigonometric Function7/1 -> Product27/2  "sin(3wt)"
  Math Function45/1 -> Add53/1
  ex/1 -> Math Function24/1
  Add27/1 -> Math Function34/1, Product50/1  "ZFC"
  Product5/1 -> Add38/2  "r/2"
  Product62/1 -> Add38/1  "r*sin(3wt)/2"
  Constant24/1 -> Math Function45/2
  Product57/1 -> Trigonometric Function12/1, Product29/2, Trigonometric Function11/1
  Product63/1 -> Product3/2, Product1/2  "1/2"
  Constant/1 -> Product63/2
  Constant19/1 -> Product62/2, Product5/1  "2"
  Math Function39/1 -> Add35/1  "10_exp(-100Dfc/r)"
  Product1/1 -> Product2/2, Add27/3  "z4/2"
  Product50/1 -> Product40/1  "Nfc"
  Constant1/1 -> Product63/1
  In1/1 -> Add27/2  "z0 - z + delta"
  Product48/1 -> Product66/2
  Product55/1 -> Add38/4  "r*sin(wt)"
  Product54/1 -> Add21/1  "r*cos(3wt)"
  Product4/1 -> Add27/4  "r*sqrt(3)/2"
  Sqrt14/1 -> Product3/1, Product2/1  "sqrt(3)"
  Product3/1 -> Product46/2, Product4/2  "sqrt(3)/2"

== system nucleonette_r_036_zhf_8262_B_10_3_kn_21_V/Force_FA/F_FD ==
  In1 : Inport
  In2 : Inport  Port=2
  Add21 : Sum
  Add27 : Sum  Inputs=-+++
  Add32 : Sum  Inputs=+++
  Add35 : Sum
  Add38 : Sum  Inputs=+++-
  Add53 : Sum
  C_100_1 : Constant  Value=-100
  C_10_1 : Constant  Value=10
  C_10_11_2 : Constant  Value=1E-21
  Clock1 : Clock
  Constant : Constant
  Constant1 : Constant  Value=2
  Constant13 : Constant  Value=3
  Constant15 : Constant  Value=1.0E-3
  Constant19 : Constant  Value=2
  Constant24 : Constant  Value=3
  Constant26 : Constant  Value=3
  Math Function{17,24,34,36} (4 alike) : Math  Operator=square
  Math Function35 : Math  Operator=pow
  Math Function39 : Math  Operator=pow
  Math Function45 : Math  Operator=pow
  Nfdx/Dfdx : Scope
  Omega_w1 : Constant  Value=0.00003453723537
  Product{1..4,27,54..56,66} (9 alike) : Product  Inputs=**
  Product{29,46,50,57} (4 alike) : Product
  Product40 : Product  Inputs=*/
  Product48 : Product  Inputs=/**
  Product5 : Product  Inputs=/*
  Product62 : Product  Inputs=*/
  Product63 : Product  Inputs=/*
  Product65 : Product  Inputs=*/*
  Sqrt10 : Sqrt
  Sqrt14 : Sqrt
  Trigonometric Function11 : Trigonometry
  Trigonometric Function12 : Trigonometry  Operator=cos
  Trigonometric Function7 : Trigonometry
  Trigonometric Function8 : Trigonometry  Operator=cos
  ex : Constant  Value=1.602176565
  kFDx : Constant  Value=66.535517341
  mFAx : Constant  Value=999.755388642
  rx1 : Constant  Value=0.36373
  Out1 : Outport
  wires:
  Product54/1 -> Add21/1  "r*cos(3wt)"
  Product55/1 -> Add38/4  "r*sin(wt)"
  Product48/1 -> Product66/2
  In1/1 -> Add27/2  "z0 - z + delta"
  Product3/1 -> Product46/2, Product4/2  "sqrt(3)/2"
  Sqrt14/1 -> Product3/1, Product2/1  "sqrt(3)"
  Product4/1 -> Add27/4  "r*sqrt(3)/2"
  Constant1/1 -> Product63/1
  Product50/1 -> Product40/1  "Nfd"
  Product1/1 -> Product2/2, Add27/3  "z4/2"
  Math Function39/1 -> Add35/1  "10_exp(-100Dfd/r)"
  Trigonometric Function8/1 -> Product54/2  "cos(3wt)"
  Product56/1 -> Add21/2  "r*cos(wt)"
  Math Function24/1 -> Product48/2
  rx1/1 -> Product27/1, Product5/2, Product54/1, Product4/1, Product65/2, Product56/1, Product55/1  "rx"
  Math Function35/1 -> Add53/2  "Dfd_3"
  Clock1/1 -> Product57/1
  Add21/1 -> Math Function36/1  "XFD"
  Trigonometric Function7/1 -> Product27/2  "sin(3wt)"
  kFDx/1 -> Product48/3
  Add32/1 -> Sqrt10/1  "Dfd_2"
  Product62/1 -> Add38/1  "r*sin(3wt)/2"
  Product29/1 -> Trigonometric Function8/1, Trigonometric Function7/1
  Add38/1 -> Math Function17/1  "YFD"
  Math Function36/1 -> Add32/2  "Xfd_2"
  Product5/1 -> Add38/2  "r/2"
  C_100_1/1 -> Product65/3
  Add53/1 -> Product40/2  "Dfd_B"
  Add35/1 -> Product66/1
  Math Function34/1 -> Add32/3  "Zfd_2"
  Sqrt10/1 -> Product65/1, Math Function35/1  "Dfd"
  Product65/1 -> Math Function39/2
  Constant13/1 -> Product29/1, Sqrt14/1
  C_10_11_2/1 -> Add35/2
  Product66/1 -> Product50/2  "kn_Dfd"
  Product2/1 -> Add38/3  "z4*sqrt(3)/2"
  Add27/1 -> Math Function34/1, Product50/1  "ZFD"
  Constant15/1 -> Math Function45/1
  Product40/1 -> Nfdx/Dfdx/1, Out1/1  "nfd/dfd"
  Trigonometric Function12/1 -> Product56/2  "cos(wt)"
  Trigonometric Function11/1 -> Product55/2  "sin(wt)"
  ex/1 -> Math Function24/1
  Product27/1 -> Product46/1, Product62/1  "r*sin(3wt)"
  Math Function17/1 -> Add32/1  "Yfd_2"
  In2/1 -> Product1/1  "z4"
  Constant24/1 -> Math Function45/2
  mFAx/1 -> Product48/1  "mx"
  Product46/1 -> Add27/1  "r*sin(3wt)*sqrt(3)/2"
  Constant26/1 -> Math Function35/2
  Math Function45/1 -> Add53/1
  Constant/1 -> Product63/2
  Constant19/1 -> Product62/2, Product5/1  "2"
  Omega_w1/1 -> Product57/2
  C_10_1/1 -> Math Function39/1
  Product63/1 -> Product3/2, Product1/2  "1/2"
  Product57/1 -> Trigonometric Function12/1, Product29/2, Trigonometric Function11/1

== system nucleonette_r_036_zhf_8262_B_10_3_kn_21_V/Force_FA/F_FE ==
  In1 : Inport
  In2 : Inport  Port=2
  Add21 : Sum  Inputs=-+
  Add27 : Sum  Inputs=++++
  Add32 : Sum  Inputs=+++
  Add35 : Sum
  Add38 : Sum  Inputs=-++-
  Add53 : Sum
  C_100_1 : Constant  Value=-100
  C_10_1 : Constant  Value=10
  C_10_11_2 : Constant  Value=1E-21
  Clock1 : Clock
  Constant : Constant
  Constant1 : Constant  Value=2
  Constant13 : Constant  Value=3
  Constant15 : Constant  Value=1.0E-3
  Constant19 : Constant  Value=2
  Constant2 : Constant  Value=0.86602
  Constant24 : Constant  Value=3
  Constant26 : Constant  Value=3
  Math Function{17,24,34,36} (4 alike) : Math  Operator=square
  Math Function35 : Math  Operator=pow
  Math Function39 : Math  Operator=pow
  Math Function45 : Math  Operator=pow
  Nfex/Dfex : Scope
  Omega_w1 : Constant  Value=0.00003453723537
  Product{1..4,27,54..56,66} (9 alike) : Product  Inputs=**
  Product{29,46,50,57} (4 alike) : Product
  Product40 : Product  Inputs=*/
  Product48 : Product  Inputs=/**
  Product5 : Product  Inputs=/*
  Product62 : Product  Inputs=*/
  Product63 : Product  Inputs=/*
  Product65 : Product  Inputs=*/*
  Sqrt10 : Sqrt
  Sqrt14 : Sqrt
  Trigonometric Function11 : Trigonometry
  Trigonometric Function12 : Trigonometry  Operator=cos
  Trigonometric Function7 : Trigonometry
  Trigonometric Function8 : Trigonometry  Operator=cos
  ex : Constant  Value=1.602176565
  kFDx : Constant  Value=66.535517341
  mFAx : Constant  Value=999.755388642
  rx1 : Constant  Value=0.36373
  Out1 : Outport
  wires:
  Product2/1 -> Add38/3  "z4*sqrt(3)/2"
  In2/1 -> Product1/1  "z4"
  Product56/1 -> Add21/2  "r*cos(wt)"
  C_10_1/1 -> Math Function39/1
  Math Function34/1 -> Add32/3  "Zfe_2"
  Clock1/1 -> Product57/1
  Trigonometric Function12/1 -> Product56/2  "cos(wt)"
  Constant26/1 -> Math Function35/2
  Product46/1 -> Add27/1  "r*sin(3wt)*sqrt(3)/2"
  Product65/1 -> Math Function39/2
  Constant15/1 -> Math Function45/1
  C_100_1/1 -> Product65/3
  Math Function36/1 -> Add32/2  "Xfe_2"
  mFAx/1 -> Product48/1  "mx"
  Add38/1 -> Math Function17/1  "YFE"
  Sqrt10/1 -> Product65/1, Math Function35/1  "Dfe"
  C_10_11_2/1 -> Add35/2
  Math Function17/1 -> Add32/1  "Yfe_2"
  Add53/1 -> Product40/2  "Dfe_B"
  kFDx/1 -> Product48/3
  Product66/1 -> Product50/2  "kn_Dfe"
  Product29/1 -> Trigonometric Function8/1, Trigonometric Function7/1
  Product27/1 -> Product46/1, Product62/1  "r*sin(3wt)"
  Add32/1 -> Sqrt10/1  "Dfe_2"
  Product40/1 -> Nfex/Dfex/1, Out1/1  "nfe/dfe"
  Omega_w1/1 -> Product57/2
  Constant13/1 -> Product29/1, Sqrt14/1
  Add35/1 -> Product66/1
  Add21/1 -> Math Function36/1  "XFE"
  Trigonometric Function11/1 -> Product55/2  "sin(wt)"
  Trigonometric Function8/1 -> Product54/2  "cos(3wt)"
  Math Function35/1 -> Add53/2  "Dfe_3"
  Math Function24/1 -> Product48/2
  rx1/1 -> Product27/1, Product5/2, Product54/1, Product4/1, Product65/2, Product56/1, Product55/1  "rx"
  Trigonometric Function7/1 -> Product27/2  "sin(3wt)"
  Math Function45/1 -> Add53/1
  ex/1 -> Math Function24/1
  Add27/1 -> Product50/1, Math Function34/1  "ZFE"
  Product5/1 -> Add38/2  "r/2"
  Product62/1 -> Add38/1  "r*sin(3wt)/2"
  Constant24/1 -> Math Function45/2
  Product57/1 -> Trigonometric Function12/1, Product29/2, Trigonometric Function11/1
  Product63/1 -> Product3/2, Product1/2  "1/2"
  Constant/1 -> Product63/2
  Constant19/1 -> Product62/2, Product5/1  "2"
  Math Function39/1 -> Add35/1  "10_exp(-100Dfe/r)"
  Product1/1 -> Product2/2, Add27/3  "z4/2"
  Product50/1 -> Product40/1  "Nfe"
  Constant1/1 -> Product63/1
  In1/1 -> Add27/2  "z0 - z + delta"
  Product48/1 -> Product66/2
  Product55/1 -> Add38/4  "r*sin(wt)"
  Product54/1 -> Add21/1  "r*cos(3wt)"
  Product4/1 -> Add27/4  "r*sqrt(3)/2"
  Sqrt14/1 -> Product3/1, Product2/1  "sqrt(3)"
  Product3/1 -> Product4/2  "sqrt(3)/2"
  Constant2/1 -> Product46/2  "sqrt(3)/2"

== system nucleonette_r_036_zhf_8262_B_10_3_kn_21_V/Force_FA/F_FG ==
  In1 : Inport
  In2 : Inport  Port=2
  Add21 : Sum  Inputs=+-+
  Add27 : Sum  Inputs=+++
  Add32 : Sum  Inputs=+++
  Add35 : Sum
  Add38 : Sum
  Add53 : Sum
  C_100_1 : Constant  Value=-100
  C_10_1 : Constant  Value=10
  C_10_11_2 : Constant  Value=1E-21
  Clock1 : Clock
  Constant13 : Constant  Value=3
  Constant15 : Constant  Value=1.0E-3
  Constant19 : Constant  Value=2
  Constant23 : Constant  Value=2
  Constant24 : Constant  Value=3
  Constant26 : Constant  Value=3
  Math Function{17,24,34,36} (4 alike) : Math  Operator=square
  Math Function35 : Math  Operator=pow
  Math Function39 : Math  Operator=pow
  Math Function45 : Math  Operator=pow
  Nfgx/Dfgx_3 : Scope
  Omega_w1 : Constant  Value=0.00003453723537
  Product{27,55..56,62,66} (5 alike) : Product  Inputs=**
  Product{29,46,50,57} (4 alike) : Product
  Product40 : Product  Inputs=*/
  Product48 : Product  Inputs=/**
  Product54 : Product  Inputs=**/
  Product63 : Product  Inputs=/*
  Product65 : Product  Inputs=*/*
  Sqrt10 : Sqrt
  Sqrt13 : Sqrt
  Sqrt14 : Sqrt
  Trigonometric Function11 : Trigonometry
  Trigonometric Function12 : Trigonometry  Operator=cos
  Trigonometric Function7 : Trigonometry
  Trigonometric Function8 : Trigonometry  Operator=cos
  ex : Constant  Value=1.602176565
  kFGx : Constant  Value=66.535517341
  mFAx : Constant  Value=999.755388642
  rx1 : Constant  Value=0.36373
  Out1 : Outport
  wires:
  Product50/1 -> Product40/1  "Nfg"
  C_10_1/1 -> Math Function39/1
  Constant26/1 -> Math Function35/2
  Product27/1 -> Add38/1  "r*sin(3wt)"
  Product46/1 -> Add27/1  "r*cos(3wt)*sqrt(3)/2"
  Product65/1 -> Math Function39/2
  Math Function36/1 -> Add32/2  "Xfg_2"
  Sqrt10/1 -> Product65/1, Math Function35/1  "Dfg"
  Math Function24/1 -> Product48/2
  mFAx/1 -> Product48/1  "mx"
  Math Function17/1 -> Add32/1  "Yfg_2"
  ex/1 -> Math Function24/1
  kFGx/1 -> Product48/3
  Add53/1 -> Product40/2  "Dfg_B"
  Add27/1 -> Product50/1, Math Function34/1  "Z2f"
  Product54/1 -> Add21/2, Product46/1  "r*cos(3wt)/2"
  C_100_1/1 -> Product65/3
  Add38/1 -> Math Function17/1  "r*sin(3wt) + r*sin(wt)"
  Product55/1 -> Add38/2  "r*sin(wt)"
  Add32/1 -> Sqrt10/1  "Dfg_2"
  Sqrt14/1 -> Product46/2  "sqrt(3)"
  Product62/1 -> Add21/1  "(z0 - z3)*sqrt(3)/2"
  Constant19/1 -> Product63/1  "2"
  Constant13/1 -> Product29/1, Sqrt14/1, Sqrt13/1
  Constant15/1 -> Math Function45/1
  Product63/1 -> Add27/2, Product62/2  "(z0 - z3)/2"
  Add35/1 -> Product66/1
  Sqrt13/1 -> Product62/1  "sqrt(3)"
  Math Function34/1 -> Add32/3  "Zfg_2"
  Product29/1 -> Trigonometric Function8/1, Trigonometric Function7/1
  Add21/1 -> Math Function36/1  "X2f"
  Constant24/1 -> Math Function45/2
  Trigonometric Function11/1 -> Product55/2  "sin(wt)"
  Constant23/1 -> Product54/3
  Trigonometric Function8/1 -> Product54/2  "cos(3wt)"
  Trigonometric Function12/1 -> Product56/2  "cos(wt)"
  rx1/1 -> Product27/1, Product54/1, Product65/2, Product56/1, Product55/1  "rx"
  Trigonometric Function7/1 -> Product27/2  "sin(3wt)"
  Math Function39/1 -> Add35/1  "10_exp(-100Dfg/r)"
  Product56/1 -> Add21/3  "r*cos(wt)"
  Product48/1 -> Product66/2
  C_10_11_2/1 -> Add35/2
  Math Function35/1 -> Add53/2  "Dfg_3"
  Product66/1 -> Product50/2  "kn_Dfg"
  In2/1 -> Product63/2
  In1/1 -> Add27/3
  Math Function45/1 -> Add53/1
  Clock1/1 -> Product57/1
  Product57/1 -> Trigonometric Function12/1, Product29/2, Trigonometric Function11/1  "angle_wt"
  Omega_w1/1 -> Product57/2
  Product40/1 -> Nfgx/Dfgx_3/1, Out1/1  "nfg/dfg_3"

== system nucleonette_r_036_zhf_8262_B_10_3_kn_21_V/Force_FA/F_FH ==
  In1 : Inport
  In2 : Inport  Port=2
  Add28 : Sum  Inputs=+-
  Add29 : Sum  Inputs=+++
  Add30 : Sum  Inputs=+--
  Add34 : Sum  Inputs=+++
  Add36 : Sum
  Add54 : Sum
  C_100_1 : Constant  Value=-100
  C_10_1 : Constant  Value=10
  C_10_11_2 : Constant  Value=1E-21
  Clock1 : Clock
  Constant{13,24..26} (4 alike) : Constant  Value=3
  Constant15 : Constant  Value=1.0E-3
  Constant19 : Constant  Value=2
  Constant23 : Constant  Value=2
  Math Function{21,24,26,31} (4 alike) : Math  Operator=square
  Math Function23 : Math  Operator=pow
  Math Function40 : Math  Operator=pow
  Math Function45 : Math  Operator=pow
  Nfhx/Dfhx_3 : Scope
  Omega_w1 : Constant  Value=0.00003453723537
  Product{27,55..56,62,67} (5 alike) : Product  Inputs=**
  Product{29,46,52,57} (4 alike) : Product
  Product47 : Product  Inputs=*/
  Product48 : Product  Inputs=/**
  Product54 : Product  Inputs=**/
  Product63 : Product  Inputs=/*
  Product64 : Product  Inputs=*/*
  Sqrt13 : Sqrt
  Sqrt14 : Sqrt
  Sqrt15 : Sqrt
  Trigonometric Function11 : Trigonometry
  Trigonometric Function12 : Trigonometry  Operator=cos
  Trigonometric Function7 : Trigonometry
  Trigonometric Function8 : Trigonometry  Operator=cos
  ex : Constant  Value=1.602176565
  kFHx : Constant  Value=66.535517341
  mFAx : Constant  Value=999.755388642
  rx1 : Constant  Value=0.36373
  Out1 : Outport
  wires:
  Product52/1 -> Product47/1  "Nfh"
  Product29/1 -> Trigonometric Function8/1, Trigonometric Function7/1
  C_10_11_2/1 -> Add36/1
  Constant13/1 -> Sqrt13/1
  Add54/1 -> Product47/2  "Dfh_B"
  Constant15/1 -> Math Function45/1
  Add29/1 -> Math Function21/1  "X3f"
  Constant25/1 -> Sqrt14/1, Product29/2
  Add34/1 -> Sqrt15/1  "Dfh_2"
  Constant24/1 -> Math Function45/2
  Trigonometric Function11/1 -> Product55/2  "sin(wt)"
  Product54/1 -> Add29/3, Product46/1  "r*cos(3wt)/2"
  Constant23/1 -> Product54/3
  Product48/1 -> Product67/2
  Trigonometric Function12/1 -> Product56/2  "cos(wt)"
  Math Function40/1 -> Add36/2  "10_exp(-100Dfh/r)"
  Product64/1 -> Math Function40/2
  Trigonometric Function7/1 -> Product27/2  "sin(3wt)"
  Product47/1 -> Out1/1, Nfhx/Dfhx_3/1  "Nfh/Dfh_3"
  ex/1 -> Math Function24/1
  Product62/1 -> Add29/1  "(z0 - z3)*sqrt(3)/2"
  Product55/1 -> Add28/2  "r*sin(wt)"
  Clock1/1 -> Product57/1
  Product27/1 -> Add28/1  "r*sin(3wt)"
  Constant26/1 -> Math Function23/2
  Sqrt14/1 -> Product46/2  "sqrt(3)"
  Sqrt13/1 -> Product62/1  "sqrt(3)"
  Product57/1 -> Trigonometric Function12/1, Trigonometric Function11/1, Product29/1
  Math Function45/1 -> Add54/1
  Math Function23/1 -> Add54/2  "Dfh_3"
  Constant19/1 -> Product63/1  "2"
  C_100_1/1 -> Product64/1
  Trigonometric Function8/1 -> Product54/2  "cos(3wt)"
  Product67/1 -> Product52/2  "kn_Dfh"
  Sqrt15/1 -> Math Function23/1, Product64/3  "Dfh"
  Product56/1 -> Add29/2  "r*cos(wt)"
  Add28/1 -> Math Function31/1  "r*sin(3wt) - r*sin(wt)"
  C_10_1/1 -> Math Function40/1
  Product46/1 -> Add30/1  "r*cos(3wt)*sqrt(3)/2"
  Product63/1 -> Add30/2, Product62/2  "(z0 - z3)/2"
  Math Function24/1 -> Product48/2
  Add36/1 -> Product67/1
  Omega_w1/1 -> Product57/2
  kFHx/1 -> Product48/3
  Math Function26/1 -> Add34/3  "Zfh_2"
  mFAx/1 -> Product48/1  "mx"
  Math Function21/1 -> Add34/2  "Xfh_2"
  Math Function31/1 -> Add34/1  "Yfh_2"
  rx1/1 -> Product56/1, Product55/1, Product27/1, Product54/1, Product64/2  "rx"
  In2/1 -> Product63/2
  Add30/1 -> Math Function26/1, Product52/1  "Z3f"
  In1/1 -> Add30/3

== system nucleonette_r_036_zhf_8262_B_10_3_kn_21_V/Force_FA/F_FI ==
  In1 : Inport
  Add31 : Sum  Inputs=+++
  Add40 : Sum
  Add51 : Sum
  C_10 : Constant  Value=10
  C_100 : Constant  Value=-100
  C_10_11 : Constant  Value=1E-21
  Clock1 : Clock
  Constant13 : Constant  Value=3
  Constant14 : Constant  Value=2
  Constant15 : Constant  Value=1.0E-3
  Constant19 : Constant  Value=2
  Constant21 : Constant  Value=1.5
  Constant24 : Constant  Value=3
  Math Function{4,27,29..30} (4 alike) : Math  Operator=square
  Math Function32 : Math  Operator=pow
  Math Function37 : Math  Operator=pow
  Math Function45 : Math  Operator=pow
  Nfix/Dfix_3 : Scope
  Omega_w1 : Constant  Value=0.00003453723537
  Product{12,20,45,57,59..60} (6 alike) : Product
  Product25 : Product  Inputs=**/
  Product26 : Product  Inputs=*/
  Product31 : Product  Inputs=/**
  Product33 : Product  Inputs=/**
  Product44 : Product  Inputs=**/
  Product58 : Product  Inputs=3
  Sqrt13 : Sqrt
  Sqrt4 : Sqrt
  Subtract3 : Sum  Inputs=-+
  Subtract4 : Sum  Inputs=-+
  Trigonometric Function10 : Trigonometry  Operator=cos
  Trigonometric Function9 : Trigonometry
  ex1 : Constant  Value=1.602176565
  keFIx_1 : Constant  Value=7.39283526
  mfx1 : Constant  Value=999.755388642
  rx1 : Constant  Value=0.36373
  sqrt(3)/2 : Constant  Value=0.86602
  Out1 : Outport
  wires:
  Subtract4/1 -> Math Function30/1
  Math Function32/1 -> Add51/2
  Add40/1 -> Product45/1  "kn_Dfi"
  Math Function45/1 -> Add51/1
  Product45/1 -> Product60/1
  Math Function4/1 -> Product31/2
  Math Function30/1 -> Add31/3
  Math Function37/1 -> Add40/1  "10_exp(-100Dfi/r)"
  Math Function29/1 -> Add31/2
  Clock1/1 -> Product57/1
  Product44/1 -> Subtract4/1  "z*sqrt(3)/2"
  sqrt(3)/2/1 -> Product58/1  "sqrt(3)/2"
  Subtract3/1 -> Math Function27/1, Product60/2  "Zfi"
  C_100/1 -> Product33/3
  Trigonometric Function10/1 -> Product58/2, Product25/1  "cos(wt)"
  Product58/1 -> Subtract3/2  "r*cos(wt)*sqrt(3)/2"
  Add51/1 -> Product26/2  "Dfi_B"
  Add31/1 -> Sqrt4/1
  C_10_11/1 -> Add40/2
  Product31/1 -> Product45/2
  Constant21/1 -> Product59/2
  Product57/1 -> Trigonometric Function9/1, Trigonometric Function10/1  "angle_wt"
  C_10/1 -> Math Function37/1
  mfx1/1 -> Product31/1  "mx"
  Constant19/1 -> Product25/3, Product44/3  "2"
  Constant13/1 -> Sqrt13/1
  Product33/1 -> Math Function37/2
  Constant15/1 -> Math Function45/1
  Product59/1 -> Subtract3/1  "3*z/2"
  Omega_w1/1 -> Product57/2
  Sqrt13/1 -> Product44/2  "sqrt(3)"
  keFIx_1/1 -> Product31/3
  ex1/1 -> Math Function4/1
  Product12/1 -> Product20/2  "r*sin(wt)"
  Math Function27/1 -> Add31/1
  Constant24/1 -> Math Function32/2, Math Function45/2
  Constant14/1 -> Product20/1
  Trigonometric Function9/1 -> Product12/1  "sin(wt)"
  Product25/1 -> Subtract4/2  "r*cos(wt)/2"
  rx1/1 -> Product33/1, Product25/2, Product12/2, Product58/3  "rx"
  Product20/1 -> Math Function29/1  "2r*sin(wt)"
  Product26/1 -> Out1/1, Nfix/Dfix_3/1  "F_FI"
  Sqrt4/1 -> Product33/2, Math Function32/1  "Dfi"
  In1/1 -> Product44/1, Product59/1  "z"
  Product60/1 -> Product26/1
